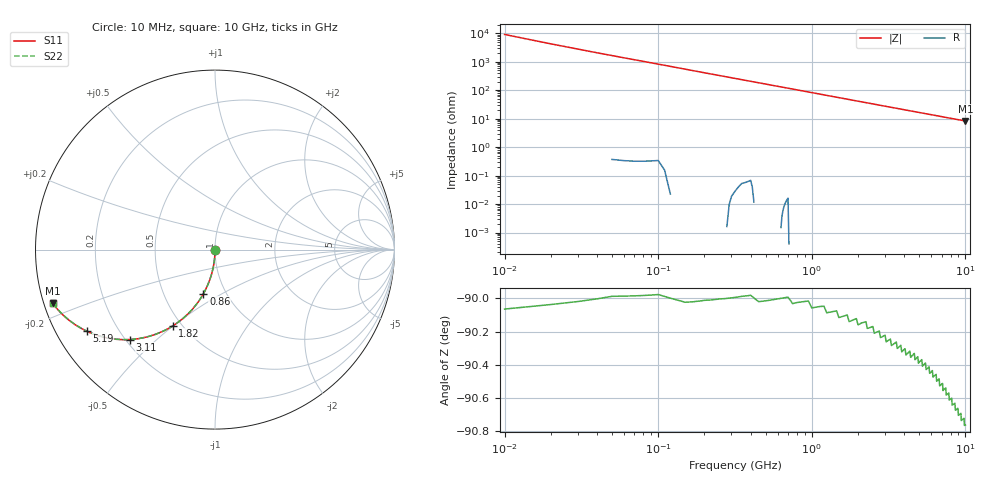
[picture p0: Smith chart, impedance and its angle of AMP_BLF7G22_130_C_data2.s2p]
! Created Thu Jul 08 13:15:04 2010
# ghz S ma R 50
! 2 Port Network Data from SP1.SP block
! freq  magS11  angS11  magS21  angS21  magS12  angS12  magS22  angS22
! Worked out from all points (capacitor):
!   1000 points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, 10 MHz to 10 GHz, reference 50 ohm
!   read as one part in shunt: C = 1.94 pF near 60 MHz
!   lowest |Z| = 8.26 ohm at 10 GHz (marker M1)
!   S11 on the Smith chart (normalised r, x): 10 MHz: 1.00, -0.01; 860 MHz: 0.78, -0.41; 1.82 GHz: 0.45, -0.50; 3.11 GHz: 0.22, -0.41; 5.19 GHz: 0.09, -0.29; 10 GHz: 0.02, -0.16
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0.01  0.002763 -90.0  1 -0.2  1 -0.2  0.002743 -89.9
0.04  0.01201 -90.6  0.9999 -0.7  0.9999 -0.7  0.01223 -90.6
0.07  0.02102 -91.2  0.9998 -1.2  0.9998 -1.2  0.02139 -91.2
0.09  0.02695 -91.6  0.9996 -1.6  0.9996 -1.6  0.0274 -91.5
0.12  0.03653 -92.1  0.9993 -2.1  0.9993 -2.1  0.03655 -92.1
0.15  0.04645 -92.6  0.9989 -2.6  0.9989 -2.6  0.04574 -92.6
0.22  0.06728 -93.8  0.9977 -3.8  0.9977 -3.8  0.06692 -93.8
0.33  0.09986 -95.7  0.9949 -5.8  0.9949 -5.8  0.1001 -95.7
0.47  0.1424 -98.1  0.9899 -8.2  0.9899 -8.2  0.1418 -98.2
0.65  0.1938 -101.2  0.9809 -11.2  0.9809 -11.2  0.1942 -101.2
0.86  0.2534 -104.7  0.9674 -14.7  0.9674 -14.7  0.2534 -104.7
1.25  0.3566 -110.8  0.9348 -20.9  0.9348 -20.9  0.3558 -110.8
1.68  0.4554 -117.0  0.8908 -27.2  0.8908 -27.2  0.4556 -117.0
1.82  0.4854 -118.9  0.8753 -29.1  0.8753 -29.1  0.4849 -118.9
2.42  0.5939 -126.3  0.806 -36.5  0.806 -36.5  0.5937 -126.3
3.11  0.6891 -133.3  0.7275 -43.6  0.7275 -43.6  0.6884 -133.3
3.34  0.7148 -135.4  0.7026 -45.7  0.7026 -45.7  0.714 -135.4
5.01  0.8385 -146.6  0.5501 -57.1  0.5501 -57.1  0.8377 -146.7
5.19  0.8467 -147.6  0.5366 -58.0  0.5366 -58.0  0.8464 -147.6
6.67  0.8992 -153.7  0.444 -64.2  0.444 -64.2  0.8988 -153.7
8.34  0.9329 -158.4  0.369 -69.1  0.369 -69.1  0.9323 -158.4
10  0.9526 -161.7  0.3149 -72.5  0.3149 -72.5  0.9519 -161.7
